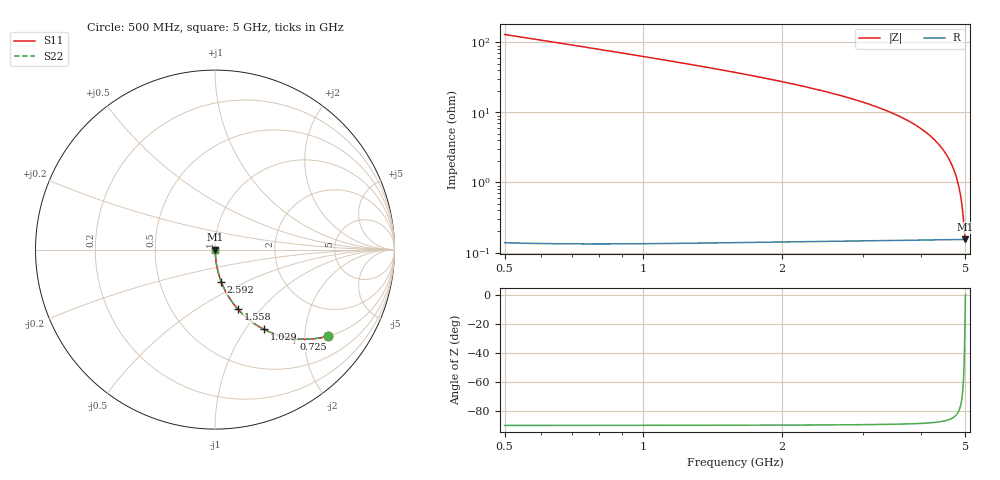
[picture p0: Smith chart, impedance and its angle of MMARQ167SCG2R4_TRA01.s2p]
! MMARQ167SCG2R4_TRA01  S-PARAMETER MODEL  ( General Type )
! Model Generated by TAIYO YUDEN Corporation (http://www.ty-top.com)
! Version 1.0
! TAIYO YUDEN Control No. 160201
! Copyright(c) 2016 TAIYO YUDEN CO.,LTD. All Rights Reserved.
! Product Description (link to TY-COMPAS)
! https://ds.yuden.co.jp/TYCOMPAS/or/detail?pn=MMARQ167SCG2R4BTRA01&u=M
! Products Name : Multilayer Ceramic Capacitors
! Characteristics :
!  Capacitance : 2.4 pF , Rated Voltage : 250V , TCC : CG / C0G
!  Case Size : 1.6 x 0.8 / 0.063 x 0.031 [mm/inch] , Thickness : 0.7 / 0.028 [mm/inch]
!  (Conditions: Temperature = 25 degC , DC Bias Current/Voltage = 0A / 0V)
! External Node Assignments :
!  1  o---| |---o  2
! GND o---------o GND
! Frequency Range : 500MHz  -  5000MHz  [ 401 STEP ]
# MHz S RI R 50
! Freq[MHz].  S11 Real  S11 Imag  S21 Real  S21 Imag  S12 Real  S12 Imag  S22 Real  S22 Imag
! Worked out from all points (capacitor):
!   401 points, 500 MHz to 5 GHz, reference 50 ohm
!   read as one part in series: C = 2.42 pF near 522.5 MHz
!   lowest |Z| = 154 mohm at 5 GHz (marker M1)
!   series resonance near 5 GHz, so ESL is about 420 pH
!   S11 on the Smith chart (normalised r, x): 500 MHz: 1.00, -2.60; 725 MHz: 1.00, -1.77; 1.029 GHz: 1.00, -1.22; 1.558 GHz: 1.00, -0.76; 2.592 GHz: 1.00, -0.37; 5 GHz: 1.00, +0.00
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500  0.6281 -0.4828  0.3719 0.4828  0.3719 0.4828  0.6281 -0.4828
725  0.4401 -0.4957  0.5599 0.4957  0.5599 0.4957  0.4401 -0.4957
871.25  0.3483 -0.4755  0.6517 0.4755  0.6517 0.4755  0.3483 -0.4755
1028.75  0.2723 -0.4441  0.7277 0.4441  0.7277 0.4441  0.2723 -0.4441
1253.75  0.1947 -0.3946  0.8053 0.3946  0.8053 0.3946  0.1947 -0.3946
1557.5  0.1274 -0.3316  0.8726 0.3316  0.8726 0.3316  0.1274 -0.3316
2007.5  0.0711 -0.2544  0.9289 0.2544  0.9289 0.2544  0.0711 -0.2544
2592.5  0.0344 -0.1784  0.9656 0.1784  0.9656 0.1784  0.0344 -0.1784
2750  0.0283 -0.1615  0.9717 0.1615  0.9717 0.1615  0.0283 -0.1615
3503.75  0.0104 -0.0942  0.9896 0.0942  0.9896 0.0942  0.0104 -0.0942
3931.25  0.00552 -0.0633  0.9945 0.0633  0.9945 0.0633  0.00552 -0.0633
4257.5  0.00329 -0.0422  0.9967 0.0422  0.9967 0.0422  0.00329 -0.0422
4426.25  0.00254 -0.0319  0.9975 0.0319  0.9975 0.0319  0.00254 -0.0319
4561.25  0.0021 -0.024  0.9979 0.024  0.9979 0.024  0.0021 -0.024
4673.75  0.00184 -0.0177  0.9982 0.0177  0.9982 0.0177  0.00184 -0.0177
4763.75  0.00169 -0.0127  0.9983 0.0127  0.9983 0.0127  0.00169 -0.0127
4831.25  0.00161 -0.00898  0.9984 0.00898  0.9984 0.00898  0.00161 -0.00898
4887.5  0.00157 -0.00595  0.9984 0.00595  0.9984 0.00595  0.00157 -0.00595
4921.25  0.00155 -0.00415  0.9985 0.00415  0.9985 0.00415  0.00155 -0.00415
4943.75  0.00154 -0.00296  0.9985 0.00296  0.9985 0.00296  0.00154 -0.00296
4977.5  0.00153 -0.00118  0.9985 0.00118  0.9985 0.00118  0.00153 -0.00118
5000  0.00153 1.61e-06  0.9985 -1.61e-06  0.9985 -1.61e-06  0.00153 1.61e-06
